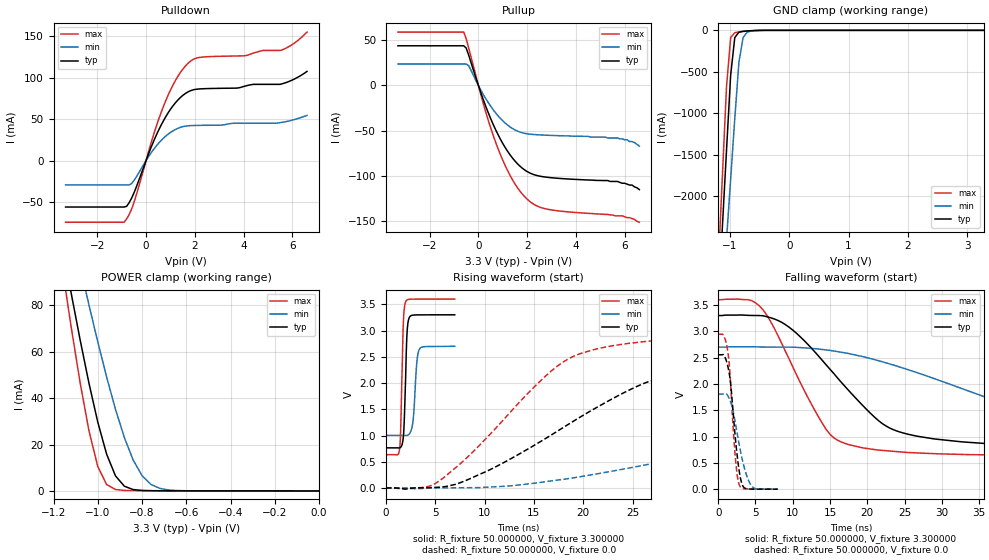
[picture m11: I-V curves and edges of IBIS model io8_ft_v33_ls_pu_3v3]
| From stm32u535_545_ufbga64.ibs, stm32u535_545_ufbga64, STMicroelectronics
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|   Model io8_ft_v33_ls_pu_3v3
[Model]  io8_ft_v33_ls_pu_3v3
Model_type I/O
Polarity   Non-Inverting
Enable   Active-Low
Vinl =   0.990000V
Vinh =   2.310000V
Vmeas =  1.650000V
Cref =   50.000000pF
Rref =   100.000000M
Vref =   0.0V
C_comp   3.252200pF   3.221000pF   3.293600pF
[Temperature Range]   25.000000   0.140000k   -40.000000
[Pullup Reference]   3.300000V   2.700000V   3.600000V
[Pulldown Reference]   0.0V   0.0V   0.0V
[POWER Clamp Reference]   3.300000V   2.700000V   3.600000V
[GND Clamp Reference]   0.0V   0.0V   0.0V
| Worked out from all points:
|   slope of the pulldown table from 0 to 0.495 V, typ, clamps not added: 14 ohm
|   slope of the pullup table from 0 to 0.495 V, typ, clamps not added: 13.7 ohm
|   GND clamp passes 1 mA (typ) near -0.51 V on its own axis
|   POWER clamp passes 1 mA (typ) near -0.85 V on its own axis
|   rising waveform, R_fixture 50.000000, V_fixture 3.300000: 20-80 % time 245ps typ, 338ps min, 228ps max; typ from 0.765 V to 3.3 V
|   rising waveform, R_fixture 50.000000, V_fixture 0.0: 20-80 % time 14.7ns typ, 31.3ns min, 9.35ns max; typ from 0.001 V to 2.55 V
|   falling waveform, R_fixture 50.000000, V_fixture 3.300000: 20-80 % time 10ns typ, 23.1ns min, 6.37ns max; typ from 3.3 V to 0.765 V
|   falling waveform, R_fixture 50.000000, V_fixture 0.0: 20-80 % time 1.01ns typ, 1.54ns min, 815ps max; typ from 2.55 V to 0.001 V
[Pulldown]
|Voltage   I(typ)   I(min)   I(max)
-3.3V     -56.06mA   -29.42mA   -74.35mA
-900mV    -56.06mA   -29.42mA   -74.35mA
-700mV    -51.09mA   -29.42mA   -65.48mA
-500mV    -39.32mA   -24.2mA    -50.88mA
300mV     22.62mA    13.13mA    30.42mA
800mV     52.54mA    29.36mA    71.75mA
1.3V      72.91mA    38.82mA    101.4mA
1.8V      84.02mA    42.13mA    119.4mA
2.3V      86.61mA    42.5mA     124.8mA
5.5V      91.96mA    45.75mA    132.9mA
6.1V      98.6mA     49.6mA     142.1mA
6.6V      107.6mA    54.5mA     155mA
[Pullup]
|Voltage   I(typ)   I(min)   I(max)
-3.3V     43.79mA    23.73mA    58.94mA
-600mV    43.79mA    23.73mA    58.94mA
-500mV    41.28mA    23.73mA    51.52mA
-400mV    33.57mA    21.9mA     41.51mA
300mV     -22.93mA   -14.5mA    -29.27mA
800mV     -54.04mA   -33.36mA   -69.41mA
1.4V      -80.24mA   -47.59mA   -104.2mA
1.7V      -89.03mA   -51.43mA   -116.5mA
2.1V      -96.56mA   -53.74mA   -127.9mA
3V        -101.9mA   -55.18mA   -137.5mA
5.7V      -106mA     -58mA      -144mA
6.6V      -115mA     -67mA      -151mA
[GND_clamp]
|Voltage   I(typ)   I(min)   I(max)
-3.3V     -9.848A    -9.957A    -9.458A
-1.2V     -3.312A    -4.013A    -2.863A
-1.13V    -2.381A    -3.274A    -1.769A
-1.06V    -1.452A    -2.535A    -684.7mA
-990mV    -542.9mA   -1.798A    -88.02mA
-920mV    -87.11mA   -1.064A    -28.44mA
-850mV    -22.1mA    -382.4mA   -19.61mA
-780mV    -11.97mA   -86.98mA   -13.71mA
-710mV    -7.619mA   -22.26mA   -8.745mA
-640mV    -4.493mA   -7.773mA   -4.817mA
-360mV    -31.22uA   -172.6uA   -8.607uA
3.28V     0A         15.66nA    -5.841nA
[POWER_clamp]
|Voltage   I(typ)   I(min)   I(max)
-3.28V    1.355A     1.167A     1.665A
-1.16V    105.8mA    131.6mA    95.87mA
-1.12V    85.09mA    114mA      70.46mA
-1.08V    65.2mA     96.88mA    46.75mA
-1.04V    46.48mA    80.2mA     25.96mA
-1V       29.64mA    64.18mA    10.49mA
-960mV    15.81mA    49.06mA    2.744mA
-920mV    6.482mA    35.16mA    613.3uA
-840mV    578.4uA    13.29mA    138.7uA
-760mV    94.46uA    2.808mA    98.68uA
-640mV    40.58uA    159.2uA    60uA
0V        0A         19.29nA    0A
[Ramp]
| variable   typ   min   max
dV/dt_r  1.53214/14.64507n   1.08405/31.24370n   1.76624/9.33613n
dV/dt_f  1.52094/10.01383n   1.01832/23.08099n   1.77907/6.35820n
R_load = 50.000000
[Rising Waveform]
R_fixture= 50.000000
V_fixture= 3.300000
V_fixture_min= 2.700000
V_fixture_max= 3.600000
|time   V(typ)   V(min)   V(max)
0s        765.1mV    1.003V     634.9mV
1.387ns   764.6mV    1.003V     738.4mV
1.499ns   776.3mV    1.003V     1.11V
1.766ns   963.1mV    1.002V     3.119V
2.004ns   2.115V     1.001V     3.548V
2.13ns    2.899V     1.002V     3.58V
2.298ns   3.207V     1.016V     3.593V
2.733ns   3.293V     1.25V      3.599V
3.363ns   3.299V     2.631V     3.6V
6.979ns   3.3V       2.7V       3.6V
[Rising Waveform]
R_fixture= 50.000000
V_fixture= 0.0
V_fixture_min= 0.0
V_fixture_max= 0.0
|time   V(typ)   V(min)   V(max)
0s        826.3uV    846.9uV    871.5uV
5.506ns   16.02mV    2.464mV    146.4mV
10.51ns   344.9mV    17.93mV    1.015V
18.52ns   1.216V     179.5mV    2.463V
25.53ns   1.943V     411.8mV    2.775V
29.53ns   2.183V     559.3mV    2.842V
40.54ns   2.424V     979.2mV    2.914V
55.56ns   2.513V     1.45V      2.938V
75.08ns   2.545V     1.679V     2.944V
249.2ns   2.554V     1.808V     2.945V
[Falling Waveform]
R_fixture= 50.000000
V_fixture= 3.300000
V_fixture_min= 2.700000
V_fixture_max= 3.600000
|time   V(typ)   V(min)   V(max)
0s        3.3V       2.7V       3.6V
5.005ns   3.3V       2.705V     3.542V
6.507ns   3.278V     2.701V     3.311V
9.009ns   3.128V     2.7V       2.622V
15.02ns   2.276V     2.637V     1.04V
21.52ns   1.301V     2.441V     743mV
29.03ns   954.2mV    2.099V     675mV
43.54ns   820.9mV    1.418V     642.7mV
62.06ns   780.9mV    1.154V     636.2mV
249.2ns   765.1mV    1.003V     634.9mV
[Falling Waveform]
R_fixture= 50.000000
V_fixture= 0.0
V_fixture_min= 0.0
V_fixture_max= 0.0
|time   V(typ)   V(min)   V(max)
0s        2.554V     1.808V     2.945V
720.7ps   2.555V     1.808V     2.918V
1.281ns   2.343V     1.778V     2.624V
1.65ns    2.035V     1.662V     2.026V
2.306ns   965.1mV    1.254V     596.3mV
2.595ns   582.5mV    1.02V      222.9mV
2.819ns   344.6mV    847.6mV    83.09mV
3.347ns   49.48mV    496.7mV    12.52mV
4.533ns   1.963mV    50.45mV    4.383mV
7.976ns   826.3uV    846.9uV    871.5uV
